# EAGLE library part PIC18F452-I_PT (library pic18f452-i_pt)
PIC18F452-I/PT, 8 bit PIC Microcontroller 40MHz 32 kB Flash, 1536 B RAM, I2C 44-Pin TQFP Source: Datasheet
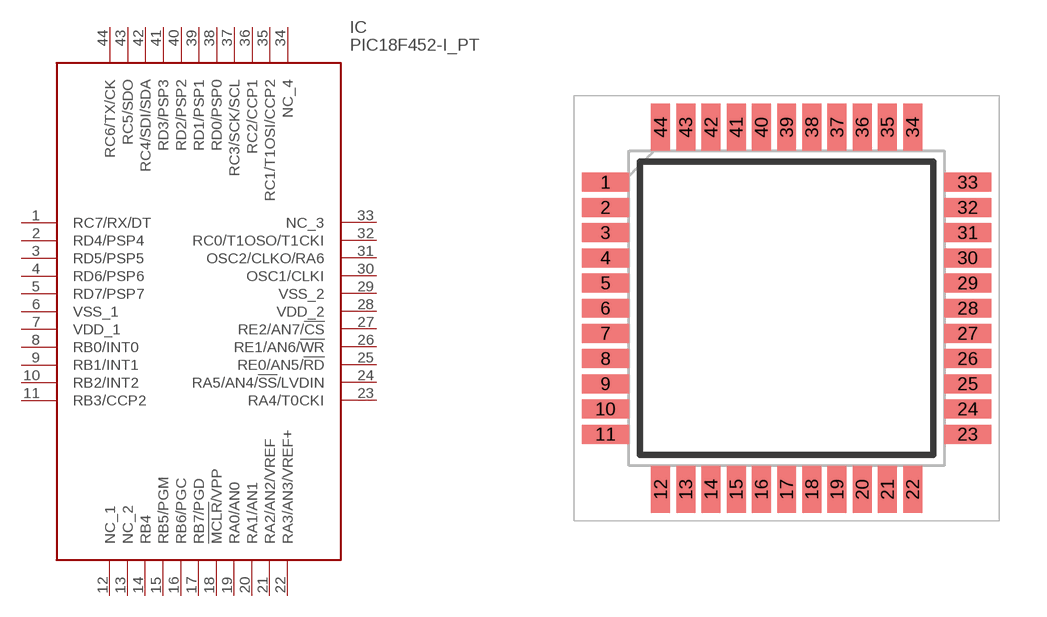
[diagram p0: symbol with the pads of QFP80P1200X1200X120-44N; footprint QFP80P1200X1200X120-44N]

Designator prefix IC

## PIC18F452-I_PT (Description: PIC18F452-I/PT, 8 bit PIC Microcontroller 40MHz 32 kB Flash, 1536 B RAM, I2C 44-Pin TQFP; Height: 1.2mm; Manufacturer_Name: Microchip; Manufacturer_Part_Number: pic18f452-i/pt; Mouser_Part_Number: 579-PIC18F452-I/PT; Mouser_Price-Stock: https://www.mouser.co.uk/ProductDetail/Microchip-Technology-Atmel/PIC18F452-I-PT?qs=6pREnGtJ7gHitcySzJWWPQ%3D%3D)  [QFP80P1200X1200X120-44N]
1  RC7/RX/DT
2  RD4/PSP4
3  RD5/PSP5
4  RD6/PSP6
5  RD7/PSP7
6  VSS_1
7  VDD_1
8  RB0/INT0
9  RB1/INT1
10  RB2/INT2
11  RB3/CCP2
12  NC_1
13  NC_2
14  RB4
15  RB5/PGM
16  RB6/PGC
17  RB7/PGD
18  !MCLR!/VPP
19  RA0/AN0
20  RA1/AN1
21  RA2/AN2/VREF
22  RA3/AN3/VREF+
23  RA4/T0CKI
24  RA5/AN4/!SS!/LVDIN
25  RE0/AN5/!RD
26  RE1/AN6/!WR
27  RE2/AN7/!CS
28  VDD_2
29  VSS_2
30  OSC1/CLKI
31  OSC2/CLKO/RA6
32  RC0/T1OSO/T1CKI
33  NC_3
34  NC_4
35  RC1/T1OSI/CCP2
36  RC2/CCP1
37  RC3/SCK/SCL
38  RD0/PSP0
39  RD1/PSP1
40  RD2/PSP2
41  RD3/PSP3
42  RC4/SDI/SDA
43  RC5/SDO
44  RC6/TX/CK

## Footprint QFP80P1200X1200X120-44N (pad centres in mm)
TQFP-44(H=1.2mm)
smd 1.5 x 0.6: 1 -5.75,4; 2 -5.75,3.2; 3 -5.75,2.4; 4 -5.75,1.6; 5 -5.75,0.8; 6 -5.75,0; 7 -5.75,-0.8; 8 -5.75,-1.6; 9 -5.75,-2.4; 10 -5.75,-3.2; 11 -5.75,-4; 23 5.75,-4; 24 5.75,-3.2; 25 5.75,-2.4; 26 5.75,-1.6; 27 5.75,-0.8; 28 5.75,0; 29 5.75,0.8; 30 5.75,1.6; 31 5.75,2.4; 32 5.75,3.2; 33 5.75,4
smd 0.6 x 1.5: 12 -4,-5.75; 13 -3.2,-5.75; 14 -2.4,-5.75; 15 -1.6,-5.75; 16 -0.8,-5.75; 17 0,-5.75; 18 0.8,-5.75; 19 1.6,-5.75; 20 2.4,-5.75; 21 3.2,-5.75; 22 4,-5.75; 34 4,5.75; 35 3.2,5.75; 36 2.4,5.75; 37 1.6,5.75; 38 0.8,5.75; 39 0,5.75; 40 -0.8,5.75; 41 -1.6,5.75; 42 -2.4,5.75; 43 -3.2,5.75; 44 -4,5.75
